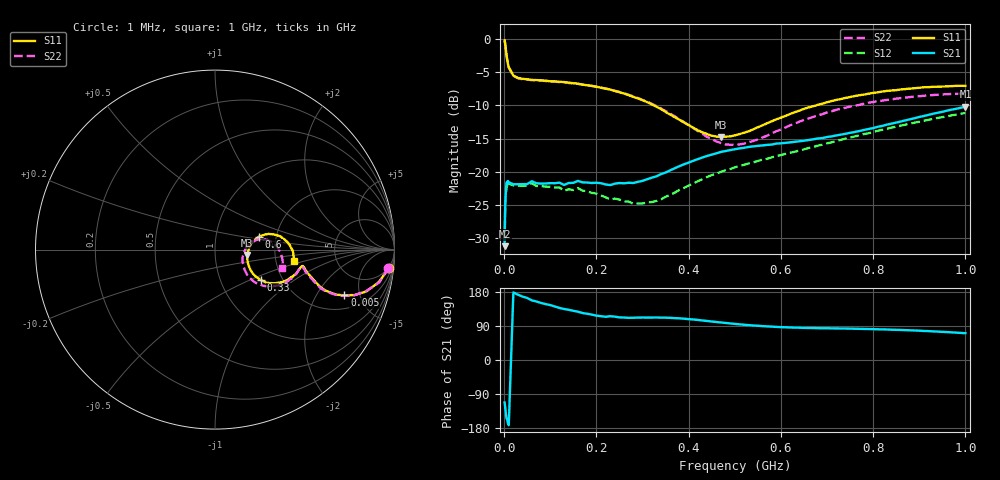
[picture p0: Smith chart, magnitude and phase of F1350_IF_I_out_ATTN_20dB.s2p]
! S-parameters for IF_I+ & IF_I- IDT F1350 DPD Demodulator
! Date Measured:  2015-11-25  RGG
!  Port 1 = Pin 19 = IF_I+
!  Port 2 = Pin 20 = IF_I-
! State: 20 dB attenuation (Gain = Gmax - 20 dB)
! IF Frequency:  1 MHz to 1000 MHz
! RF_INX, RF_INY, IF_Q+, and IF_Q- terminated
! 2300 MHz, 0 dBm signal applied to LO_IN
! Vcc = +5.00 Volts  Icc = approx 275 mA.
! NOTES:  The device was measured on a custom printed circuit evaluation board with individual 50 ohm
!  microstrip lines to the RF and LO pins. The IF outputs are normally connected to balun
!  transformers, which convert the balanced IF output signals to single ended (SE) 50 ohm signals
!  for normal test purposes. For these measurements, to measure the IFI+ and IFI- output SE s-parameters,
!  the chokes associated with the IFI+ and IFI- outputs were removed and a pair of pigtailed
!  50 ohm coaxial lines were soldered to the PCB at these points. 5.00 volt bias was provided
!  to these pins via external bias tees. Data was collected using a calibrated vector
!  network analyzer.  The pigtailed 50 ohm coaxial lines were de-embedded using reference
!  plane extensions. 100 ohm microstrip lines of length 386 mils and 218 mils for the IF_I+ and IF_I-
!  signals, respectively, were de-embedded using Agilent ADS, yielding the reference plane at the IC edge.
!  Only IFI+ and IFI- outputs were measured. IF_Q+ and IF_Q- should be identical.
!  This data is single-ended relative to ports IF_I+ and IF_I- (reference impedance = 50 ohms)
!  Common mode or differential S-parameters may be extracted from this data with a linear simulator.
# mhz S db R 50
! freq  dbS11  angS11  dbS21  angS21  dbS12  angS12  dbS22  angS22
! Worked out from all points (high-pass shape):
!   109 points, 1 MHz to 1 GHz, reference 50 ohm
!   highest |S21| = -10.19 dB at 1 GHz (marker M1); lowest = -31.2 dB at 1 MHz (marker M2)
!   |S21| within 3 dB of the highest: 813.2 MHz to end of sweep
!   lowest |S11| = -14.8 dB at 470 MHz (marker M3), VSWR 1.45, Z = 71.8 - j4.36 ohm
!   |S11| at or under -10 dB: 324.1 MHz to 676.2 MHz (352.2 MHz wide, 70.4 % of centre)
!   |S22| runs from -15.9 to -0.3 dB; largest |S21 - S12| = 0.066
!   S11 on the Smith chart (normalised r, x): 1 MHz: 4, -18; 5 MHz: 2.91, -3.58; 330 MHz: 1.56, -0.59; 600 MHz: 1.62, +0.25; 1 GHz: 2.52, -0.39
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1  -0.22 -6.1  -31.21 -112.1  -30.58 -109.1  -0.27 -6.0
2  -0.62 -11.1  -26.05 -122.0  -26.49 -116.9  -0.60 -11.4
3  -1.15 -15.4  -23.91 -132.8  -23.83 -130.6  -1.19 -15.4
5  -2.32 -19.5  -21.69 -153.4  -22.56 -151.1  -2.36 -19.8
8  -3.70 -20.3  -21.39 -166.3  -21.44 -166.3  -3.74 -20.5
9  -4.02 -19.7  -21.53 -168.7  -21.75 -166.8  -4.06 -20.1
20  -5.52 -14.1  -21.90 178.3  -22.05 178.7  -5.57 -14.5
40  -6.00 -10.8  -21.86 167.2  -22.12 168.3  -6.06 -11.1
60  -6.17 -10.9  -21.43 157.4  -21.73 158.5  -6.20 -11.3
130  -6.50 -15.9  -22.00 134.5  -22.88 136.3  -6.48 -16.6
160  -6.74 -18.9  -21.38 127.4  -22.47 129.7  -6.76 -20.4
170  -6.88 -19.6  -21.60 123.9  -22.85 126.3  -6.87 -21.1
280  -8.72 -30.6  -21.70 111.5  -24.83 114.7  -8.64 -33.7
330  -10.21 -33.5  -20.69 112.2  -24.40 122.3  -10.10 -38.3
340  -10.56 -33.6  -20.36 111.7  -24.15 123.3  -10.47 -38.8
420  -13.76 -25.0  -18.10 105.7  -21.42 124.1  -13.86 -34.7
470  -14.77 -9.2  -17.01 99.1  -20.02 119.4  -15.68 -21.4
510  -14.34 3.3  -16.49 94.1  -19.13 115.9  -15.89 -7.5
600  -11.86 16.4  -15.71 86.8  -17.49 109.2  -13.65 11.2
670  -10.14 16.3  -15.12 84.4  -16.26 104.9  -11.74 13.0
840  -7.76 5.2  -12.75 79.9  -13.35 92.6  -9.10 1.3
1000  -7.06 -8.1  -10.19 70.7  -11.15 78.5  -8.20 -15.1
